(* Logix 5000 DataType export; software revision 16.04 *)

TYPE AKD_Status :   // All connections to the drive ethernet module are established and data is successfully transferring.
STRUCT
   Profile_In_Progress : BOOL;   // Profile Move In Progress
   Block_In_Execution : BOOL;   // Block In Execution
   On_Target_Position : BOOL;   // On Target Position (1=Current Position Equals Last Target Position)
   General_Fault : BOOL;   // General Fault
   Current_Direction : BOOL;   // Current Motor Direction (0=Reverse, 1=Forward)
   Home_Level : BOOL;   // Level of Home Input
   Reg_Level : BOOL;   // Level of Registration Input
   Enable : BOOL;   // State of Enable Output
   Fault_Input_Fault : BOOL;   // Fault Input Active
   Fwd_Limit : BOOL;   // Forward Input Active
   Rev_Limit : BOOL;   // Reverse Input Active
   Positive_Limit : BOOL;   // Positive Software Limit Exceeded
   Negative_Limit : BOOL;   // Negative Software Limit Exceeded
   FE_Fault : BOOL;   // Following Error Fault
   Block_Fault : BOOL;   // Block Execution Fault
   Load_Complete : BOOL;   // Command Message Successfully Loaded
END_STRUCT
END_TYPE

TYPE AKD_Axis :   // Axis Data:
STRUCT
   Control : AKD_Control;   // Control bits to send to the drive
   Status : AKD_Status;   // Status bits received from the drive
   Input : AB:ETHERNET_MODULE_SINT_64Bytes:I:0;   // Data from the drive
   Output : AB:ETHERNET_MODULE_SINT_64Bytes:O:0;   // Data to the drive
   ResponseMsgType : SINT;   // Response type contained in latest IO response from drive. Used to check for errors
   CommandTimeout : INT;   // Time to allow for command response from drive. Dependent on scan rate and communicaiton rate
   PositionFeedback : DINT;   // Actual Position Value
   VelocityFeedback : DINT;   // Actual Velocity Value
END_STRUCT
END_TYPE

TYPE AKD_Control :   // Send Explicit Message
STRUCT
   Load_Data_Start_Profile : BOOL;   // Load Command Data / Start Profile Move
   Start_Block : BOOL;   // Execute Command block or block chain
   Incremental : BOOL;   // Incremental Position (0=Absolute, 1=Incremental)
   Direction : BOOL;   // Direction in Velocity Mode (0=Reverse, 1=Forward)
   Smooth_Stop : BOOL;   // Smooth / Controlled Stop w/ Deceleration
   Hard_Stop : BOOL;   // Hard / Immediate Stop
   Reg_Arm : BOOL;   // Arm the Registration Input
   Enable : BOOL;   // Enable Output
END_STRUCT
END_TYPE
